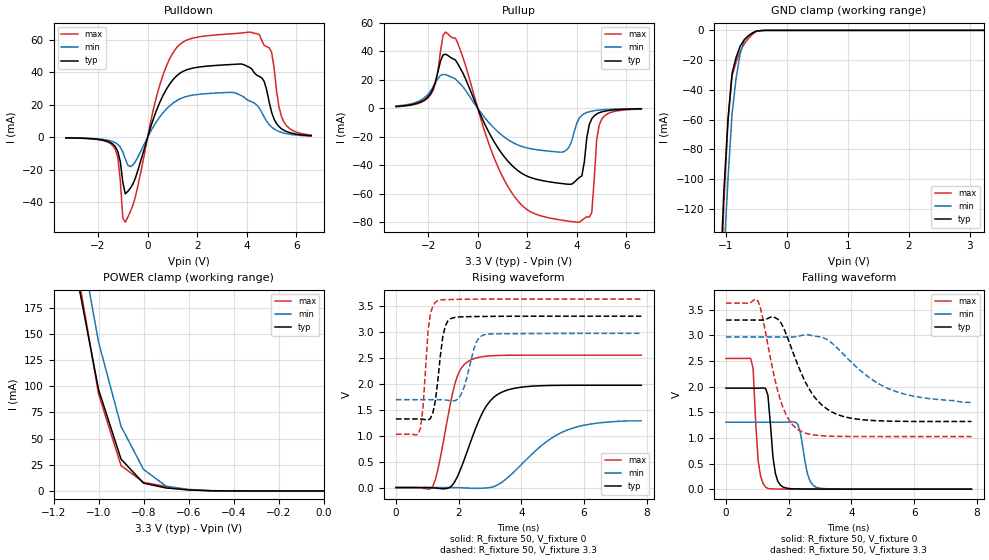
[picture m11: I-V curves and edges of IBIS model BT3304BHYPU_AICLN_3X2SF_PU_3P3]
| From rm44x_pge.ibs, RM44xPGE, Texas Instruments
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|   Model Cell BT3304BHYPU_AICLN_3X2SF_PU_3P3
|BT3304BHYPU_AICLN_3X2SF_PU_3P3
[Model]   BT3304BHYPU_AICLN_3X2SF_PU_3P3
Model_type   I/O
Polarity   Non-Inverting
Enable   Active-Low
Vinl =  1.15
Vinh =  1.55
Cref =  15.0001pF
Rref =  101.0000M
Vref =  0V
Vmeas =  1.65
C_comp   1.2p   1.2p   1.2p
[Model Spec]
Vinl   1.15   1.02   1.28
Vinh   1.55   1.45   1.65
[Temperature Range]   25   155   -40
[Voltage Range]   3.3   2.97   3.63
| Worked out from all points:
|   slope of the pulldown table from 0 to 0.495 V, typ, clamps not added: 22.9 ohm
|   slope of the pullup table from 0 to 0.495 V, typ, clamps not added: 26.9 ohm
|   GND clamp passes 1 mA (typ) near -0.53 V on its own axis
|   POWER clamp passes 1 mA (typ) near -0.60 V on its own axis
|   rising waveform, R_fixture 50, V_fixture 0: 20-80 % time 801ps typ, 1.49ns min, 507ps max; typ from 0 V to 1.97 V
|   rising waveform, R_fixture 50, V_fixture 3.3: 20-80 % time 228ps typ, 333ps min, 181ps max; typ from 1.32 V to 3.3 V
|   falling waveform, R_fixture 50, V_fixture 0: 20-80 % time 181ps typ, 234ps min, 147ps max; typ from 1.97 V to 0 V
|   falling waveform, R_fixture 50, V_fixture 3.3: 20-80 % time 942ps typ, 1.62ns min, 605ps max; typ from 3.3 V to 1.32 V
[POWER_clamp]
|   voltage   I(typ)   I(min)   I(max)
-3.3V     3.99A      4.579A     4.788A
-1.1V     209.6mA    262.2mA    219.1mA
-1.067V   172.1mA    222.3mA    177mA
-1.033V   134.5mA    182.3mA    134.9mA
-1V       96.98mA    142.4mA    92.77mA
-900mV    30.42mA    61.81mA    24.22mA
-800mV    7.461mA    20.58mA    8.236mA
-700mV    2.845mA    4.596mA    4.214mA
-600mV    944uA      1.092mA    1.45mA
-500mV    147.5uA    237.2uA    206.1uA
0V        457.2pA    5.75nA     459.6pA
[Pulldown]
|   voltage   I(typ)   I(min)   I(max)
-3.3V     -317.2uA   -283uA     -323.2uA
-1.4V     -4.187mA   -2.645mA   -5.141mA
-1.2V     -8.732mA   -4.393mA   -12.51mA
-1V       -27.63mA   -8.973mA   -49.56mA
-900mV    -34.73mA   -13.26mA   -52.12mA
400mV     18.17mA    10.56mA    27.32mA
1.1V      36.68mA    21.82mA    53.65mA
4.1V      43.08mA    22.4mA     64.63mA
4.7V      34.41mA    12.54mA    56.53mA
5V        15.54mA    6.34mA     52.45mA
5.5V      4.314mA    2.594mA    9.388mA
6.6V      981uA      787.2uA    1.387mA
[Pullup]
|   voltage   I(typ)   I(min)   I(max)
-3.3V     1.246mA    1.609mA    1.076mA
-2V       8.232mA    9.997mA    7.367mA
-1.4V     37.5mA     23.8mA     51.32mA
-900mV    33.96mA    20.66mA    49.39mA
1.4V      -40.56mA   -23.96mA   -60.16mA
3.4V      -52.99mA   -30.87mA   -78.78mA
4V        -50.22mA   -10.35mA   -80.18mA
4.2V      -47.59mA   -4.955mA   -78.93mA
4.6V      -7.373mA   -1.996mA   -73.36mA
4.8V      -3.99mA    -1.436mA   -21.72mA
5V        -2.558mA   -1.08mA    -7.69mA
6.6V      -380.4uA   -267.9uA   -552uA
[GND_clamp]
|   voltage   I(typ)   I(min)   I(max)
-3.3V     -3.259A    -2.879A    -4.965A
-1.1V     -172mA     -209.5mA   -194.3mA
-1.033V   -107.5mA   -151.2mA   -115.7mA
-966.7mV  -59.82mA   -100mA     -61.12mA
-900mV    -29.02mA   -56.02mA   -30.7mA
-833.3mV  -18.2mA    -32.16mA   -21.26mA
-766.7mV  -10.64mA   -15.72mA   -14.06mA
-700mV    -6.323mA   -6.701mA   -9.103mA
-566.7mV  -1.777mA   -1.727mA   -2.678mA
-500mV    -473.5uA   -571uA     -709.6uA
-366.7mV  -40.38uA   -55.9uA    -61.97uA
3.233V    -1.26uA    5.628uA    -10.55uA
[Ramp]
| variable   typ   min   max
dV/dt_f   1.227312/0.9529086n  0.7926917/1.641681n   1.612216/0.6137352n
dV/dt_r   1.196553/0.8079251n  0.7933102/1.54853n   1.548881/0.5102178n
R_load = 50
[Rising Waveform]
R_fixture = 50
V_fixture = 0
V_fixture_min = 0
V_fixture_max = 0
|   time   V(typ)   V(min)   V(max)
0s        296.2uV    223.4uV    361.7uV
1.18ns    -5.368mV   218uV      30.07mV
1.336ns   -12.9mV    240.7uV    340.7mV
1.888ns   126.1mV    -770.6uV   2.014V
2.092ns   398.6mV    -4.117mV   2.306V
2.392ns   897mV      -11.7mV    2.459V
2.9ns     1.586V     -6.473mV   2.53V
3.58ns    1.883V     198.6mV    2.548V
5.392ns   1.969V     1.09V      2.551V
7.828ns   1.971V     1.284V     2.551V
[Rising Waveform]
R_fixture = 50
V_fixture = 3.3
V_fixture_min = 2.97
V_fixture_max = 3.63
|   time   V(typ)   V(min)   V(max)
0s        1.322V     1.693V     1.027V
784ps     1.321V     1.693V     1.144V
864ps     1.317V     1.693V     1.535V
1.024ns   1.299V     1.693V     3.012V
1.18ns    1.44V      1.693V     3.501V
1.336ns   2.056V     1.693V     3.599V
1.572ns   3.107V     1.687V     3.619V
1.808ns   3.266V     1.668V     3.622V
2.8ns     3.295V     2.939V     3.629V
7.828ns   3.3V       2.97V      3.63V
[Falling Waveform]
R_fixture = 50
V_fixture = 0
V_fixture_min = 0
V_fixture_max = 0
|   time   V(typ)   V(min)   V(max)
0s        1.971V     1.307V     2.551V
784ps     1.971V     1.307V     2.552V
864ps     1.971V     1.307V     2.355V
1.024ns   1.97V      1.307V     555.2mV
1.336ns   1.829V     1.307V     13.27mV
1.572ns   312.1mV    1.307V     4.298mV
1.808ns   44.96mV    1.306V     2.911mV
2.292ns   5.125mV    1.255V     1.343mV
2.9ns     2.309mV    33.02mV    589.4uV
7.828ns   313.6uV    453.6uV    384uV
[Falling Waveform]
R_fixture = 50
V_fixture = 3.3
V_fixture_min = 2.97
V_fixture_max = 3.63
|   time   V(typ)   V(min)   V(max)
0s        3.3V       2.97V      3.63V
1.024ns   3.3V       2.97V      3.668V
1.732ns   3.263V     2.97V      1.742V
1.988ns   2.912V     2.97V      1.373V
2.344ns   2.342V     2.99V      1.143V
2.9ns     1.739V     2.98V      1.051V
3.696ns   1.427V     2.662V     1.029V
4.604ns   1.343V     2.16V      1.028V
5.392ns   1.325V     1.91V      1.027V
7.828ns   1.321V     1.693V     1.027V
